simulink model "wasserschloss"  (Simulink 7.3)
settings: Solver=ode23tb  StartTime=0.0  StopTime=1000  MaxStep=0.5  RelTol=1e-3
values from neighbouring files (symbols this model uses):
  A_W = pi*5^2    (= 78.5398163397)    [dynamic_main.m]    (also in Parameter.m; Parameter_sim.m; static_main.m)
  h_W_IC = 413    [dynamic_main.m]    (also in Parameter.m; Parameter_sim.m; static_main.m)
  lambda_W = fminsearch(@(lambda_W)err_wasserschloss(lambda_W,time_bb,V_flw_T_bb,V_flw_F_bb,h_W_bb),lambda_W0)    [dynamic_main.m]    (also in Parameter.m = 10; Parameter_sim.m = 4.0738)

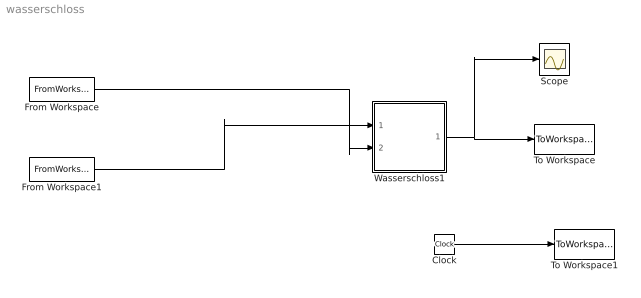
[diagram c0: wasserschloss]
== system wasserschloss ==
  Clock : Clock
  From Workspace : FromWorkspace  VariableName=[time_bb V_flw_T_bb]  SampleTime=0
  From Workspace1 : FromWorkspace  VariableName=[time_bb V_flw_F_bb]  SampleTime=0
  Scope : Scope
  To Workspace : ToWorkspace  VariableName=h_W  SampleTime=-1  SaveFormat=Array
  To Workspace1 : ToWorkspace  VariableName=time_sim  SampleTime=-1  SaveFormat=Array
  Wasserschloss1 : Subsystem
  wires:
  Wasserschloss1/1(h_W) -> To Workspace/1, Scope/1
  Clock/1 -> To Workspace1/1
  From Workspace1/1 -> Wasserschloss1/1(v_F)
  From Workspace/1 -> Wasserschloss1/2(v_T)

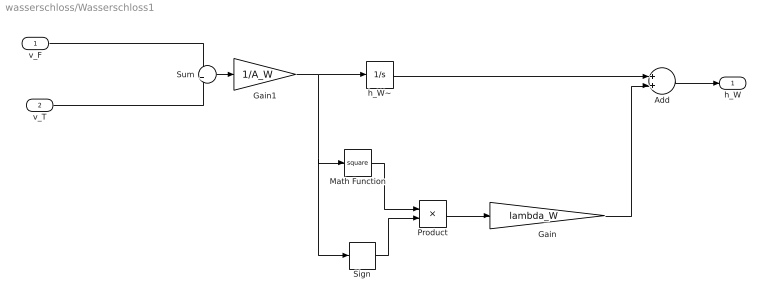
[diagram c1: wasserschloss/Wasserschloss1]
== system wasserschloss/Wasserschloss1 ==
  v_F : Inport  OutDataType=sfix(16)  OutScaling=2^0
  v_T : Inport  Port=2  OutDataType=sfix(16)  OutScaling=2^0
  Add : Sum  OutDataType=sfix(16)  OutScaling=2^-10
  Gain : Gain  Gain=lambda_W  ParameterDataType=sfix(16)  ParameterScaling=2^0  OutDataType=sfix(16)  OutScaling=2^0
  Gain1 : Gain  Gain=1/A_W  ParameterDataType=sfix(16)  ParameterScaling=2^0  OutDataType=sfix(16)  OutScaling=2^0
  Math Function : Math  Operator=square  OutDataType=sfix(16)  OutScaling=2^0
  Product : Product  OutDataType=sfix(16)  OutScaling=2^0
  Sign : Signum
  Sum : Sum  Inputs=-+  OutDataType=sfix(16)  OutScaling=2^0
  h_W~ : Integrator  InitialCondition=h_W_IC
  h_W : Outport  OutDataType=sfix(16)  OutScaling=2^0
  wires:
  Product/1 -> Gain/1
  Sum/1 -> Gain1/1
  Gain1/1 -> h_W~/1, Math Function/1, Sign/1
  Math Function/1 -> Product/1
  Sign/1 -> Product/2
  h_W~/1 -> Add/1
  Add/1 -> h_W/1
  Gain/1 -> Add/2
  v_F/1 -> Sum/1
  v_T/1 -> Sum/2
